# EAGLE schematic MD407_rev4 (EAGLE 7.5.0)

## Sheet 1 of 7: OVERVIEW
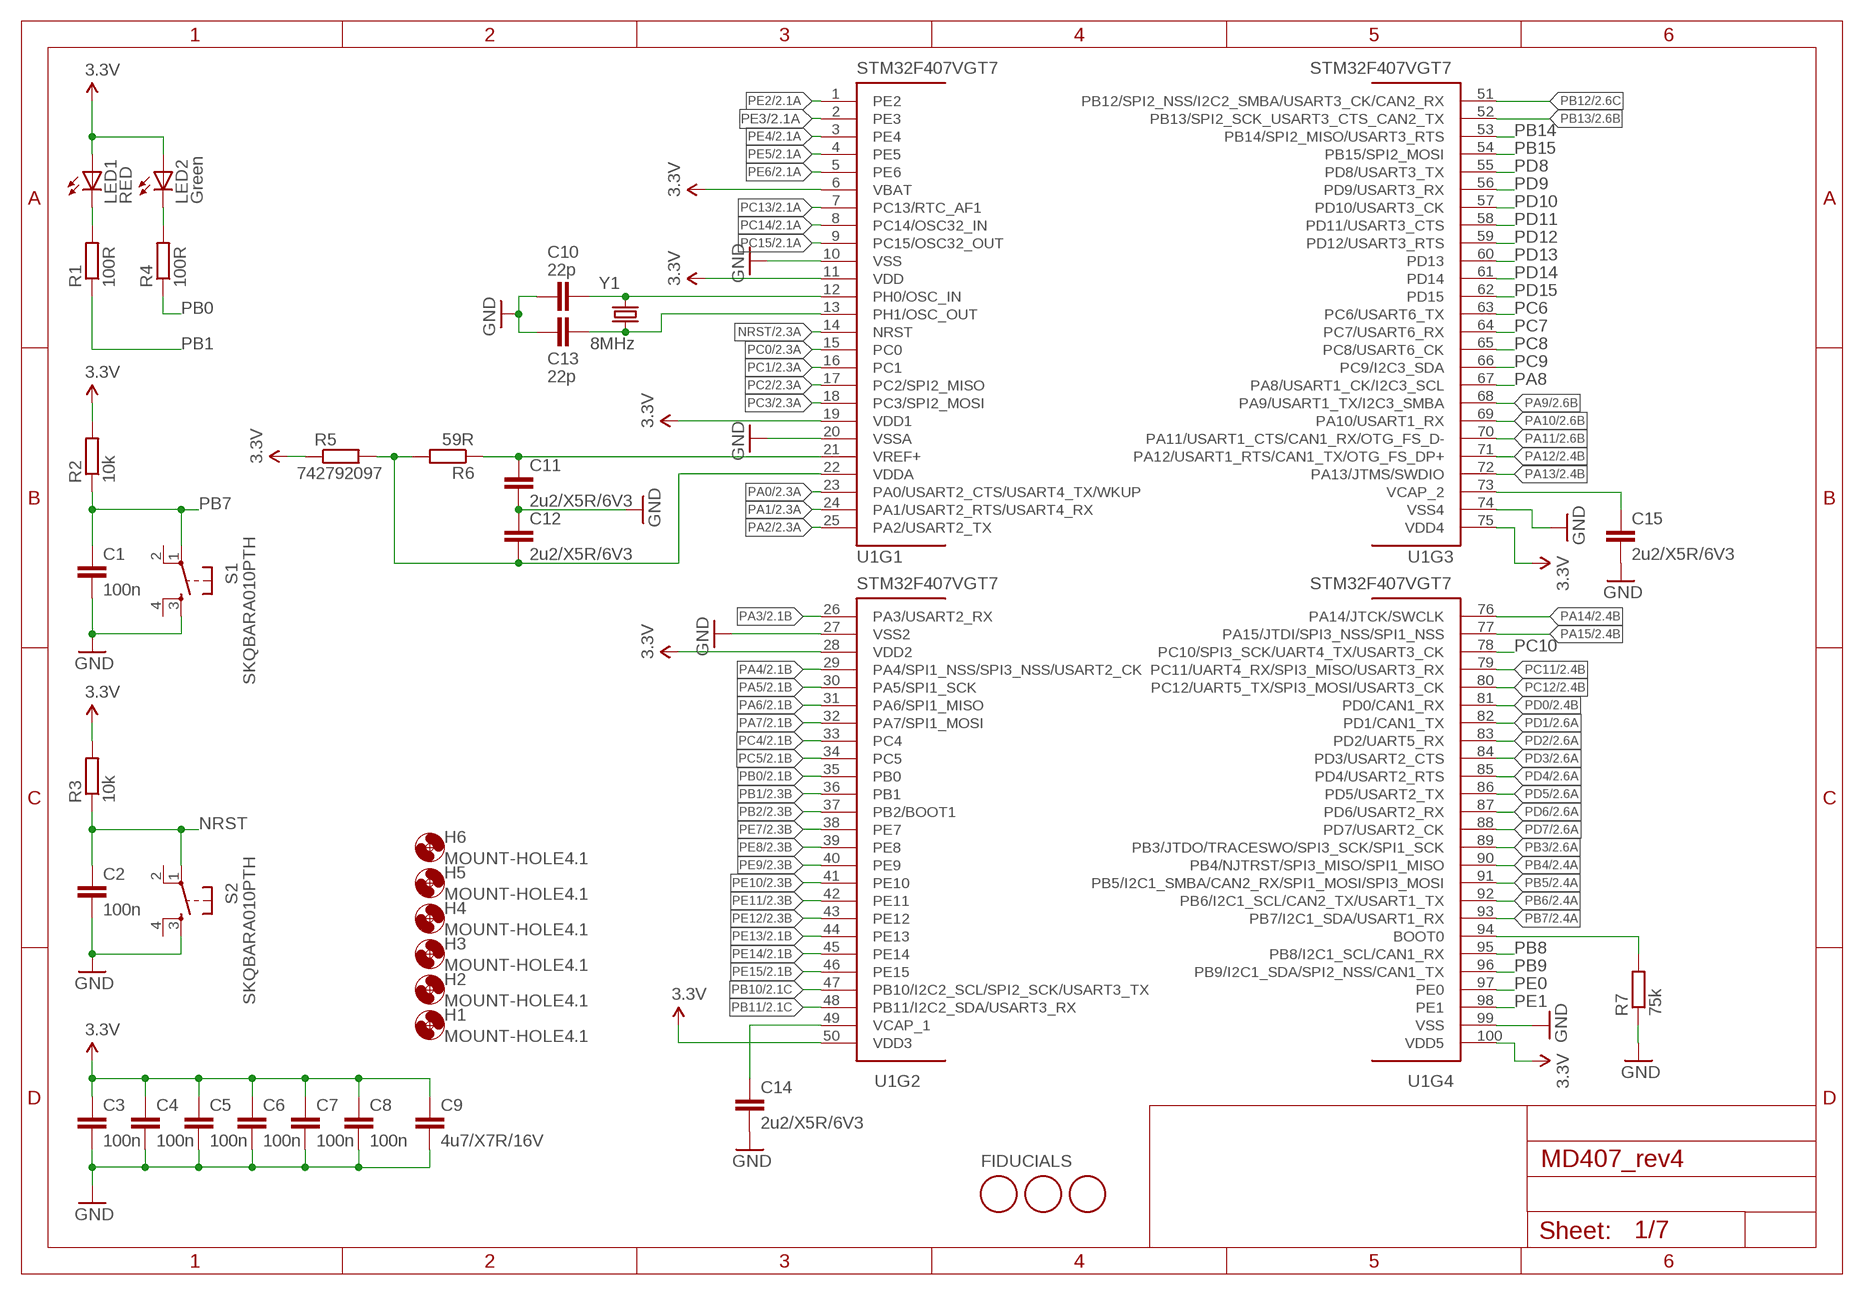
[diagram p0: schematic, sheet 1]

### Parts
C1  100n  C-EUC0603  [C0603]
C2  100n  C-EUC0603  [C0603]
C3  100n  C-EUC0603  [C0603]
C4  100n  C-EUC0603  [C0603]
C5  100n  C-EUC0603  [C0603]
C6  100n  C-EUC0603  [C0603]
C7  100n  C-EUC0603  [C0603]
C8  100n  C-EUC0603  [C0603]
C9  4u7/X7R/16V  C-EUC0805  [C0805]
C10  22p  C-EUC0603  [C0603]
C11  2u2/X5R/6V3  C-EUC0603  [C0603]
C12  2u2/X5R/6V3  C-EUC0603  [C0603]
C13  22p  C-EUC0603  [C0603]
C14  2u2/X5R/6V3  C-EUC0603  [C0603]
C15  2u2/X5R/6V3  C-EUC0603  [C0603]
H1  MOUNT-HOLE4.1  [4,1]
H2  MOUNT-HOLE4.1  [4,1]
H3  MOUNT-HOLE4.1  [4,1]
H4  MOUNT-HOLE4.1  [4,1]
H5  MOUNT-HOLE4.1  [4,1]
H6  MOUNT-HOLE4.1  [4,1]
LED1  RED  LED0603  [LED-0603]
LED2  Green  LED0603  [LED-0603]
R1  100R  R-EU_R0603  [R0603]
R2  10k  R-EU_R0603  [R0603]
R3  10k  R-EU_R0603  [R0603]
R4  100R  R-EU_R0603  [R0603]
R5  742792097  R-EU_R0805  [R0805]
R6  59R  R-EU_R0603  [R0603]
R7  75k  R-EU_R0603  [R0603]
S1  SKQBARA010PTH  [TACTILE-PTH]
S2  SKQBARA010PTH  [TACTILE-PTH]
U1  STM32F407VGT7  [LQFP100]
U$1  FIDUCIAL  [FIDUCIAL_1MM]
U$2  FIDUCIAL  [FIDUCIAL_1MM]
U$3  FIDUCIAL  [FIDUCIAL_1MM]
Y1  8MHz  7B-8.000MAAJ-T  [CRYSTAL-SMD-5X3]

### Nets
3.3V: C3.1 C4.1 C5.1 C6.1 C7.1 C8.1 C9.1 LED1.A LED2.A R2.2 R3.2 R5.1 U1.6(VBAT) U1.11(VDD) U1.19(VDD1) U1.28(VDD2) U1.50(VDD3) U1.75(VDD4) U1.100(VDD5) ; also sheet 2,3,4,5,6,7
GND: C1.2 C2.2 C3.2 C4.2 C5.2 C6.2 C7.2 C8.2 C9.2 C10.1 C11.2 C12.1 C13.2 C14.2 C15.2 R7.1 S1.3 S2.3 U1.10(VSS) U1.20(VSSA) U1.27(VSS2) U1.74(VSS4) U1.99(VSS) ; also sheet 2,3,4,5,6,7
N$9: LED2.C R4.2
N$11: R7.2 U1.94(BOOT0)
N$27: C15.1 U1.73(VCAP_2)
N$43: C12.2 R5.2 R6.2 U1.22(VDDA)
N$45: C10.2 U1.12(PH0/OSC_IN) Y1.3
N$49: C13.1 U1.13(PH1/OSC_OUT) Y1.1
N$63: C11.1 R6.1 U1.21(VREF+)
N$77: C14.1 U1.49(VCAP_1)
N$87: LED1.C R1.2
NRST: C2.1 R3.1 S2.1 U1.14(NRST) ; also sheet 2,6
PA0: U1.23(PA0/USART2_CTS/USART4_TX/WKUP) ; also sheet 2
PA1: U1.24(PA1/USART2_RTS/USART4_RX) ; also sheet 2,6
PA2: U1.25(PA2/USART2_TX) ; also sheet 2,6
PA3: U1.26(PA3/USART2_RX) ; also sheet 2
PA4: U1.29(PA4/SPI1_NSS/SPI3_NSS/USART2_CK) ; also sheet 2
PA5: U1.30(PA5/SPI1_SCK) ; also sheet 2,3
PA6: U1.31(PA6/SPI1_MISO) ; also sheet 2
PA7: U1.32(PA7/SPI1_MOSI) ; also sheet 2,6
PA8: U1.67(PA8/USART1_CK/I2C3_SCL) ; also sheet 2
PA9: U1.68(PA9/USART1_TX/I2C3_SMBA) ; also sheet 2,4
PA10: U1.69(PA10/USART1_RX) ; also sheet 2,4
PA11: U1.70(PA11/USART1_CTS/CAN1_RX/OTG_FS_D-) ; also sheet 2,4
PA12: U1.71(PA12/USART1_RTS/CAN1_TX/OTG_FS_DP+) ; also sheet 2,4
PA13: U1.72(PA13/JTMS/SWDIO) ; also sheet 2
PA14: U1.76(PA14/JTCK/SWCLK) ; also sheet 2
PA15: U1.77(PA15/JTDI/SPI3_NSS/SPI1_NSS) ; also sheet 2
PB0: R4.1 U1.35(PB0) ; also sheet 2
PB1: R1.1 U1.36(PB1) ; also sheet 2
PB2: U1.37(PB2/BOOT1) ; also sheet 2
PB3: U1.89(PB3/JTDO/TRACESWO/SPI3_SCK/SPI1_SCK) ; also sheet 2
PB4: U1.90(PB4/NJTRST/SPI3_MISO/SPI1_MISO) ; also sheet 2
PB5: U1.91(PB5/I2C1_SMBA/CAN2_RX/SPI1_MOSI/SPI3_MOSI) ; also sheet 2,7
PB6: U1.92(PB6/I2C1_SCL/CAN2_TX/USART1_TX) ; also sheet 2,7
PB7: C1.1 R2.1 S1.1 U1.93(PB7/I2C1_SDA/USART1_RX) ; also sheet 2
PB8: U1.95(PB8/I2C1_SCL/CAN1_RX) ; also sheet 2,7
PB9: U1.96(PB9/I2C1_SDA/SPI2_NSS/CAN1_TX) ; also sheet 2,7
PB10: U1.47(PB10/I2C2_SCL/SPI2_SCK/USART3_TX) ; also sheet 2
PB11: U1.48(PB11/I2C2_SDA/USART3_RX) ; also sheet 2,6
PB12: U1.51(PB12/SPI2_NSS/I2C2_SMBA/USART3_CK/CAN2_RX) ; also sheet 2,6
PB13: U1.52(PB13/SPI2_SCK_USART3_CTS_CAN2_TX) ; also sheet 2,6
PB14: U1.53(PB14/SPI2_MISO/USART3_RTS) ; also sheet 2
PB15: U1.54(PB15/SPI2_MOSI) ; also sheet 2
PC0: U1.15(PC0) ; also sheet 2
PC1: U1.16(PC1) ; also sheet 2,6
PC2: U1.17(PC2/SPI2_MISO) ; also sheet 2
PC3: U1.18(PC3/SPI2_MOSI) ; also sheet 2
PC4: U1.33(PC4) ; also sheet 2,6
PC5: U1.34(PC5) ; also sheet 2,6
PC6: U1.63(PC6/USART6_TX) ; also sheet 2
PC7: U1.64(PC7/USART6_RX) ; also sheet 2
PC8: U1.65(PC8/USART6_CK) ; also sheet 2
PC9: U1.66(PC9/I2C3_SDA) ; also sheet 2
PC10: U1.78(PC10/SPI3_SCK/UART4_TX/USART3_CK) ; also sheet 2,3
PC11: U1.79(PC11/UART4_RX/SPI3_MISO/USART3_RX) ; also sheet 2,3
PC12: U1.80(PC12/UART5_TX/SPI3_MOSI/USART3_CK) ; also sheet 2,3
PC13: U1.7(PC13/RTC_AF1) ; also sheet 2
PC14: U1.8(PC14/OSC32_IN) ; also sheet 2
PC15: U1.9(PC15/OSC32_OUT) ; also sheet 2
PD0: U1.81(PD0/CAN1_RX) ; also sheet 2
PD1: U1.82(PD1/CAN1_TX) ; also sheet 2
PD2: U1.83(PD2/UART5_RX) ; also sheet 2
PD3: U1.84(PD3/USART2_CTS) ; also sheet 2,3
PD4: U1.85(PD4/USART2_RTS) ; also sheet 2
PD5: U1.86(PD5/USART2_TX) ; also sheet 2
PD6: U1.87(PD6/USART2_RX) ; also sheet 2
PD7: U1.88(PD7/USART2_CK) ; also sheet 2
PD8: U1.55(PD8/USART3_TX) ; also sheet 2
PD9: U1.56(PD9/USART3_RX) ; also sheet 2
PD10: U1.57(PD10/USART3_CK) ; also sheet 2
PD11: U1.58(PD11/USART3_CTS) ; also sheet 2
PD12: U1.59(PD12/USART3_RTS) ; also sheet 2
PD13: U1.60(PD13) ; also sheet 2
PD14: U1.61(PD14) ; also sheet 2
PD15: U1.62(PD15) ; also sheet 2
PE0: U1.97(PE0) ; also sheet 2
PE1: U1.98(PE1) ; also sheet 2
PE2: U1.1(PE2) ; also sheet 2
PE3: U1.2(PE3) ; also sheet 2
PE4: U1.3(PE4) ; also sheet 2
PE5: U1.4(PE5) ; also sheet 2
PE6: U1.5(PE6) ; also sheet 2
PE7: U1.38(PE7) ; also sheet 2
PE8: U1.39(PE8) ; also sheet 2
PE9: U1.40(PE9) ; also sheet 2
PE10: U1.41(PE10) ; also sheet 2
PE11: U1.42(PE11) ; also sheet 2
PE12: U1.43(PE12) ; also sheet 2
PE13: U1.44(PE13) ; also sheet 2
PE14: U1.45(PE14) ; also sheet 2
PE15: U1.46(PE15) ; also sheet 2
Unconnected: S1.2 S1.4 S2.2 S2.4

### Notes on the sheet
- FIDUCIALS

## Sheet 2 of 7: EXP-headers
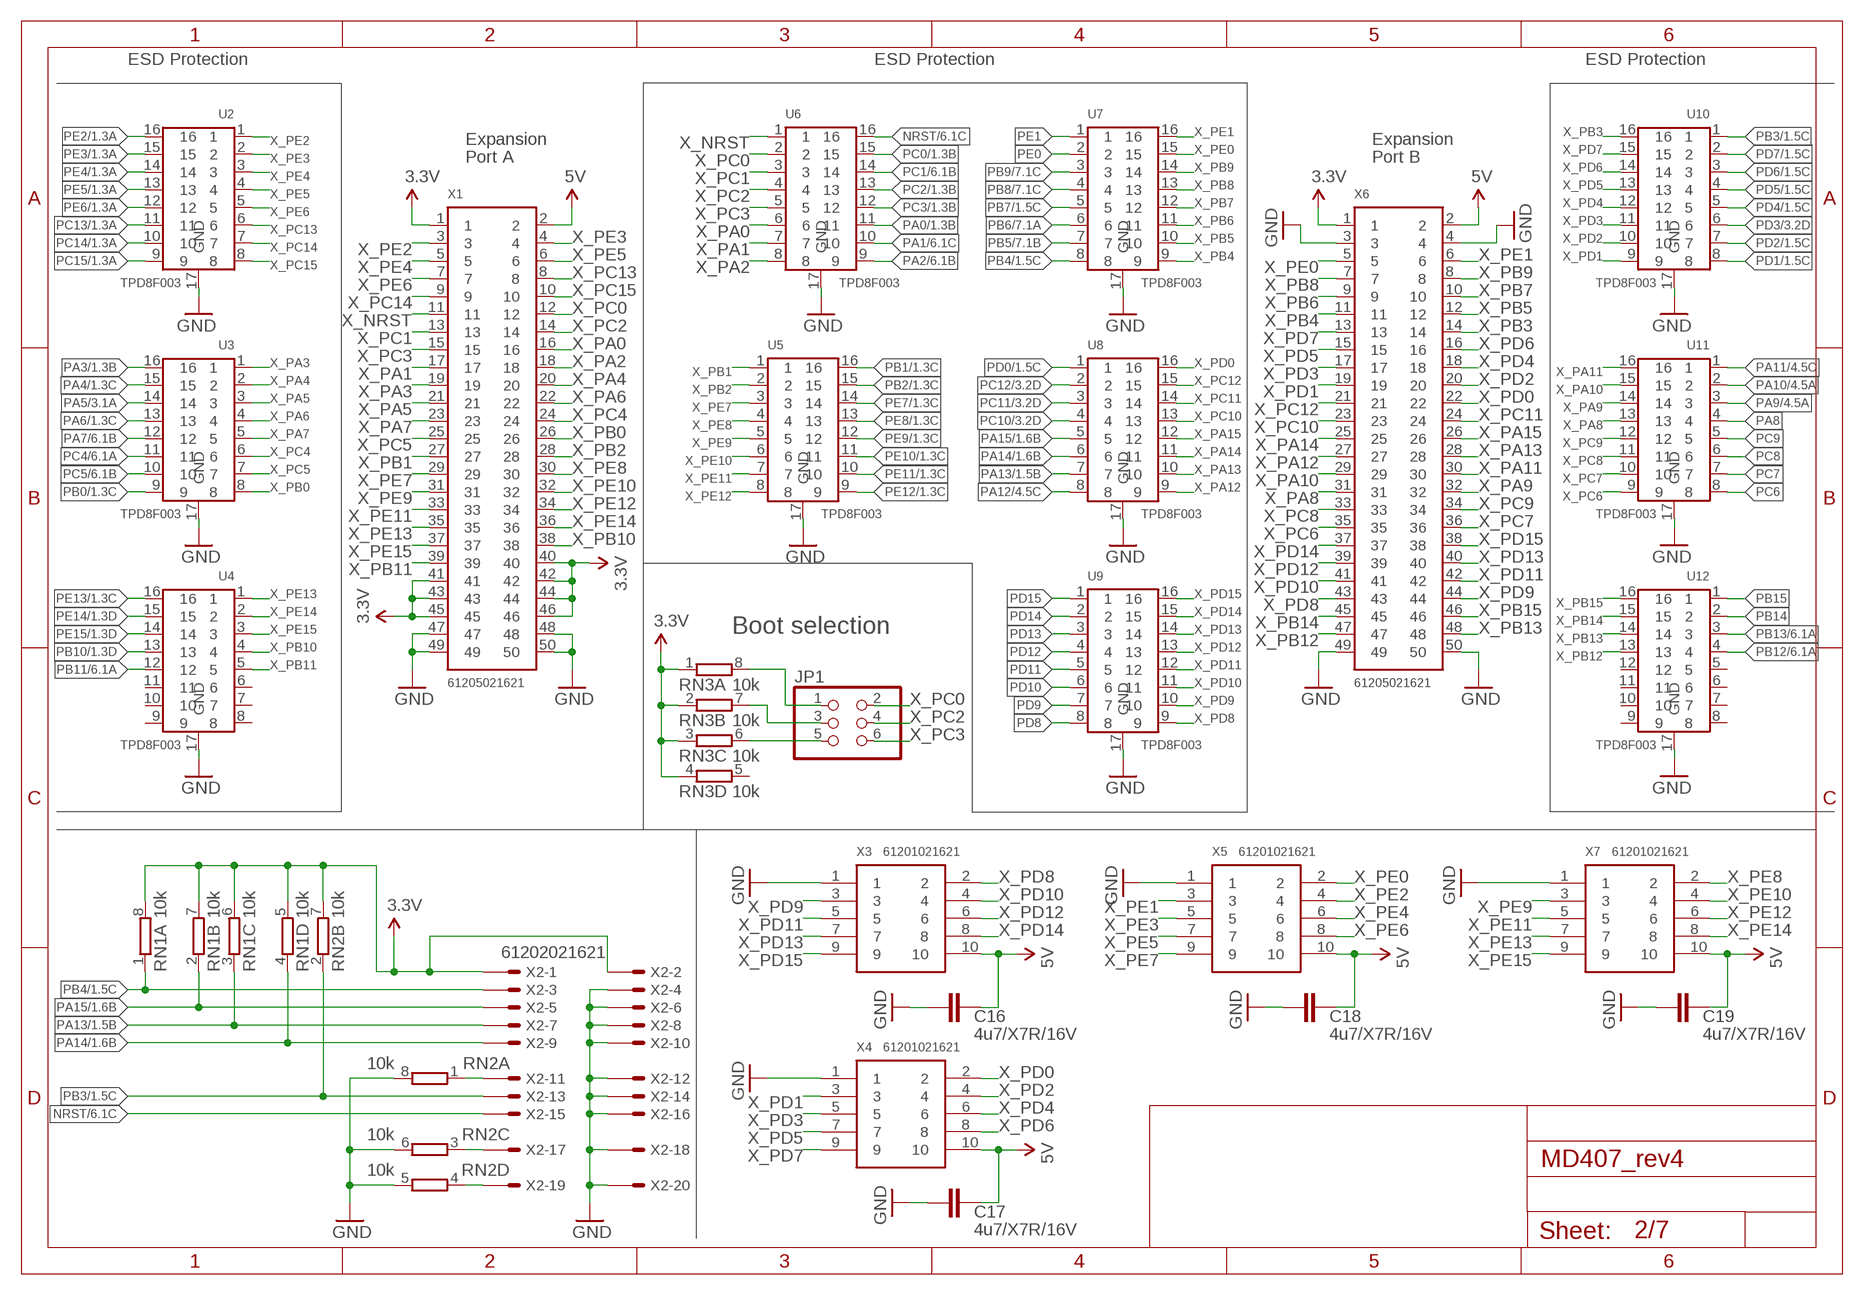
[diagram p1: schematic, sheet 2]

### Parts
C16  4u7/X7R/16V  C-EUC0805  [C0805]
C17  4u7/X7R/16V  C-EUC0805  [C0805]
C18  4u7/X7R/16V  C-EUC0805  [C0805]
C19  4u7/X7R/16V  C-EUC0805  [C0805]
JP1  PINHD-2X3  [2X03]
RN1  10k  4R-NCAY16  [CAY16]
RN2  10k  4R-NCAY16  [CAY16]
RN3  10k  4R-NCAY16  [CAY16]
U2  TPD8F003  [16-WFDFN]
U3  TPD8F003  [16-WFDFN]
U4  TPD8F003  [16-WFDFN]
U5  TPD8F003  [16-WFDFN]
U6  TPD8F003  [16-WFDFN]
U7  TPD8F003  [16-WFDFN]
U8  TPD8F003  [16-WFDFN]
U9  TPD8F003  [16-WFDFN]
U10  TPD8F003  [16-WFDFN]
U11  TPD8F003  [16-WFDFN]
U12  TPD8F003  [16-WFDFN]
X1  61205021621  [057-050-1]
X2  61202021621  [057-020-1]
X3  61201021621  [057-010-1]
X4  61201021621  [057-010-1]
X5  61201021621  [057-010-1]
X6  61205021621  [057-050-1]
X7  61201021621  [057-010-1]

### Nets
3.3V: RN1.5 RN1.6 RN1.7 RN1.8 RN2.7 RN3.1 RN3.2 RN3.3 RN3.4 X1.1 X1.40 X1.41 X1.42 X1.43 X1.44 X1.45 X1.46 X2.1 X2.2 X6.1 ; also sheet 1,3,4,5,6,7
5V: C16.1 C17.1 C18.1 C19.1 X1.2 X3.10 X4.10 X5.10 X6.2 X7.10 ; also sheet 3,4,5,7
GND: C16.2 C17.2 C18.2 C19.2 RN2.5 RN2.6 RN2.8 U2.17(GND) U3.17(GND) U4.17(GND) U5.17(GND) U6.17(GND) U7.17(GND) U8.17(GND) U9.17(GND) U10.17(GND) U11.17(GND) U12.17(GND) X1.47 X1.48 X1.49 X1.50 X2.4 X2.6 X2.8 X2.10 X2.12 X2.14 X2.16 X2.18 X2.20 X3.1 X4.1 X5.1 X6.3 X6.4 X6.49 X6.50 X7.1 ; also sheet 1,3,4,5,6,7
N$8: JP1.1 RN3.8
N$23: JP1.3 RN3.7
N$41: JP1.5 RN3.6
N$71: RN2.3 X2.17
N$96: RN2.4 X2.19
N$97: RN2.1 X2.11
NRST: U6.16 X2.15 ; also sheet 1,6
PA0: U6.11 ; also sheet 1
PA1: U6.10 ; also sheet 1,6
PA2: U6.9 ; also sheet 1,6
PA3: U3.16 ; also sheet 1
PA4: U3.15 ; also sheet 1
PA5: U3.14 ; also sheet 1,3
PA6: U3.13 ; also sheet 1
PA7: U3.12 ; also sheet 1,6
PA8: U11.4 ; also sheet 1
PA9: U11.3 ; also sheet 1,4
PA10: U11.2 ; also sheet 1,4
PA11: U11.1 ; also sheet 1,4
PA12: U8.8 ; also sheet 1,4
PA13: RN1.3 U8.7 X2.7 ; also sheet 1
PA14: RN1.4 U8.6 X2.9 ; also sheet 1
PA15: RN1.2 U8.5 X2.5 ; also sheet 1
PB0: U3.9 ; also sheet 1
PB1: U5.16 ; also sheet 1
PB2: U5.15 ; also sheet 1
PB3: RN2.2 U10.1 X2.13 ; also sheet 1
PB4: RN1.1 U7.8 X2.3 ; also sheet 1
PB5: U7.7 ; also sheet 1,7
PB6: U7.6 ; also sheet 1,7
PB7: U7.5 ; also sheet 1
PB8: U7.4 ; also sheet 1,7
PB9: U7.3 ; also sheet 1,7
PB10: U4.13 ; also sheet 1
PB11: U4.12 ; also sheet 1,6
PB12: U12.4 ; also sheet 1,6
PB13: U12.3 ; also sheet 1,6
PB14: U12.2 ; also sheet 1
PB15: U12.1 ; also sheet 1
PC0: U6.15 ; also sheet 1
PC1: U6.14 ; also sheet 1,6
PC2: U6.13 ; also sheet 1
PC3: U6.12 ; also sheet 1
PC4: U3.11 ; also sheet 1,6
PC5: U3.10 ; also sheet 1,6
PC6: U11.8 ; also sheet 1
PC7: U11.7 ; also sheet 1
PC8: U11.6 ; also sheet 1
PC9: U11.5 ; also sheet 1
PC10: U8.4 ; also sheet 1,3
PC11: U8.3 ; also sheet 1,3
PC12: U8.2 ; also sheet 1,3
PC13: U2.11 ; also sheet 1
PC14: U2.10 ; also sheet 1
PC15: U2.9 ; also sheet 1
PD0: U8.1 ; also sheet 1
PD1: U10.8 ; also sheet 1
PD2: U10.7 ; also sheet 1
PD3: U10.6 ; also sheet 1,3
PD4: U10.5 ; also sheet 1
PD5: U10.4 ; also sheet 1
PD6: U10.3 ; also sheet 1
PD7: U10.2 ; also sheet 1
PD8: U9.8 ; also sheet 1
PD9: U9.7 ; also sheet 1
PD10: U9.6 ; also sheet 1
PD11: U9.5 ; also sheet 1
PD12: U9.4 ; also sheet 1
PD13: U9.3 ; also sheet 1
PD14: U9.2 ; also sheet 1
PD15: U9.1 ; also sheet 1
PE0: U7.2 ; also sheet 1
PE1: U7.1 ; also sheet 1
PE2: U2.16 ; also sheet 1
PE3: U2.15 ; also sheet 1
PE4: U2.14 ; also sheet 1
PE5: U2.13 ; also sheet 1
PE6: U2.12 ; also sheet 1
PE7: U5.14 ; also sheet 1
PE8: U5.13 ; also sheet 1
PE9: U5.12 ; also sheet 1
PE10: U5.11 ; also sheet 1
PE11: U5.10 ; also sheet 1
PE12: U5.9 ; also sheet 1
PE13: U4.16 ; also sheet 1
PE14: U4.15 ; also sheet 1
PE15: U4.14 ; also sheet 1
X_NRST: U6.1 X1.11
X_PA0: U6.6 X1.16
X_PA1: U6.7 X1.17
X_PA2: U6.8 X1.18
X_PA3: U3.1 X1.19
X_PA4: U3.2 X1.20
X_PA5: U3.3 X1.21
X_PA6: U3.4 X1.22
X_PA7: U3.5 X1.23
X_PA8: U11.13 X6.31
X_PA9: U11.14 X6.32
X_PA10: U11.15 X6.29
X_PA11: U11.16 X6.30
X_PA12: U8.9 X6.27
X_PA13: U8.10 X6.28
X_PA14: U8.11 X6.25
X_PA15: U8.12 X6.26
X_PB0: U3.8 X1.26
X_PB1: U5.1 X1.27
X_PB2: U5.2 X1.28
X_PB3: U10.16 X6.14
X_PB4: U7.9 X6.11
X_PB5: U7.10 X6.12
X_PB6: U7.11 X6.9
X_PB7: U7.12 X6.10
X_PB8: U7.13 X6.7
X_PB9: U7.14 X6.8
X_PB10: U4.4 X1.38
X_PB11: U4.5 X1.39
X_PB12: U12.13 X6.47
X_PB13: U12.14 X6.48
X_PB14: U12.15 X6.45
X_PB15: U12.16 X6.46
X_PC0: JP1.2 U6.2 X1.12
X_PC1: U6.3 X1.13
X_PC2: JP1.4 U6.4 X1.14
X_PC3: JP1.6 U6.5 X1.15
X_PC4: U3.6 X1.24
X_PC5: U3.7 X1.25
X_PC6: U11.9 X6.35
X_PC7: U11.10 X6.36
X_PC8: U11.11 X6.33
X_PC9: U11.12 X6.34
X_PC10: U8.13 X6.23
X_PC11: U8.14 X6.24
X_PC12: U8.15 X6.21
X_PC13: U2.6 X1.8
X_PC14: U2.7 X1.9
X_PC15: U2.8 X1.10
X_PD0: U8.16 X4.2 X6.22
X_PD1: U10.9 X4.3 X6.19
X_PD2: U10.10 X4.4 X6.20
X_PD3: U10.11 X4.5 X6.17
X_PD4: U10.12 X4.6 X6.18
X_PD5: U10.13 X4.7 X6.15
X_PD6: U10.14 X4.8 X6.16
X_PD7: U10.15 X4.9 X6.13
X_PD8: U9.9 X3.2 X6.43
X_PD9: U9.10 X3.3 X6.44
X_PD10: U9.11 X3.4 X6.41
X_PD11: U9.12 X3.5 X6.42
X_PD12: U9.13 X3.6 X6.39
X_PD13: U9.14 X3.7 X6.40
X_PD14: U9.15 X3.8 X6.37
X_PD15: U9.16 X3.9 X6.38
X_PE0: U7.15 X5.2 X6.5
X_PE1: U7.16 X5.3 X6.6
X_PE2: U2.1 X1.3 X5.4
X_PE3: U2.2 X1.4 X5.5
X_PE4: U2.3 X1.5 X5.6
X_PE5: U2.4 X1.6 X5.7
X_PE6: U2.5 X1.7 X5.8
X_PE7: U5.3 X1.29 X5.9
X_PE8: U5.4 X1.30 X7.2
X_PE9: U5.5 X1.31 X7.3
X_PE10: U5.6 X1.32 X7.4
X_PE11: U5.7 X1.33 X7.5
X_PE12: U5.8 X1.34 X7.6
X_PE13: U4.1 X1.35 X7.7
X_PE14: U4.2 X1.36 X7.8
X_PE15: U4.3 X1.37 X7.9
Unconnected: RN3.5 U4.6 U4.7 U4.8 U4.9 U4.10 U4.11 U12.5 U12.6 U12.7 U12.8 U12.9 U12.10 U12.11 U12.12

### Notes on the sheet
- ESD Protection | ESD Protection | ESD Protection
- Expansion | Expansion
- Port A | Port B
- Boot selection

## Sheet 3 of 7: SOUND + JTAG
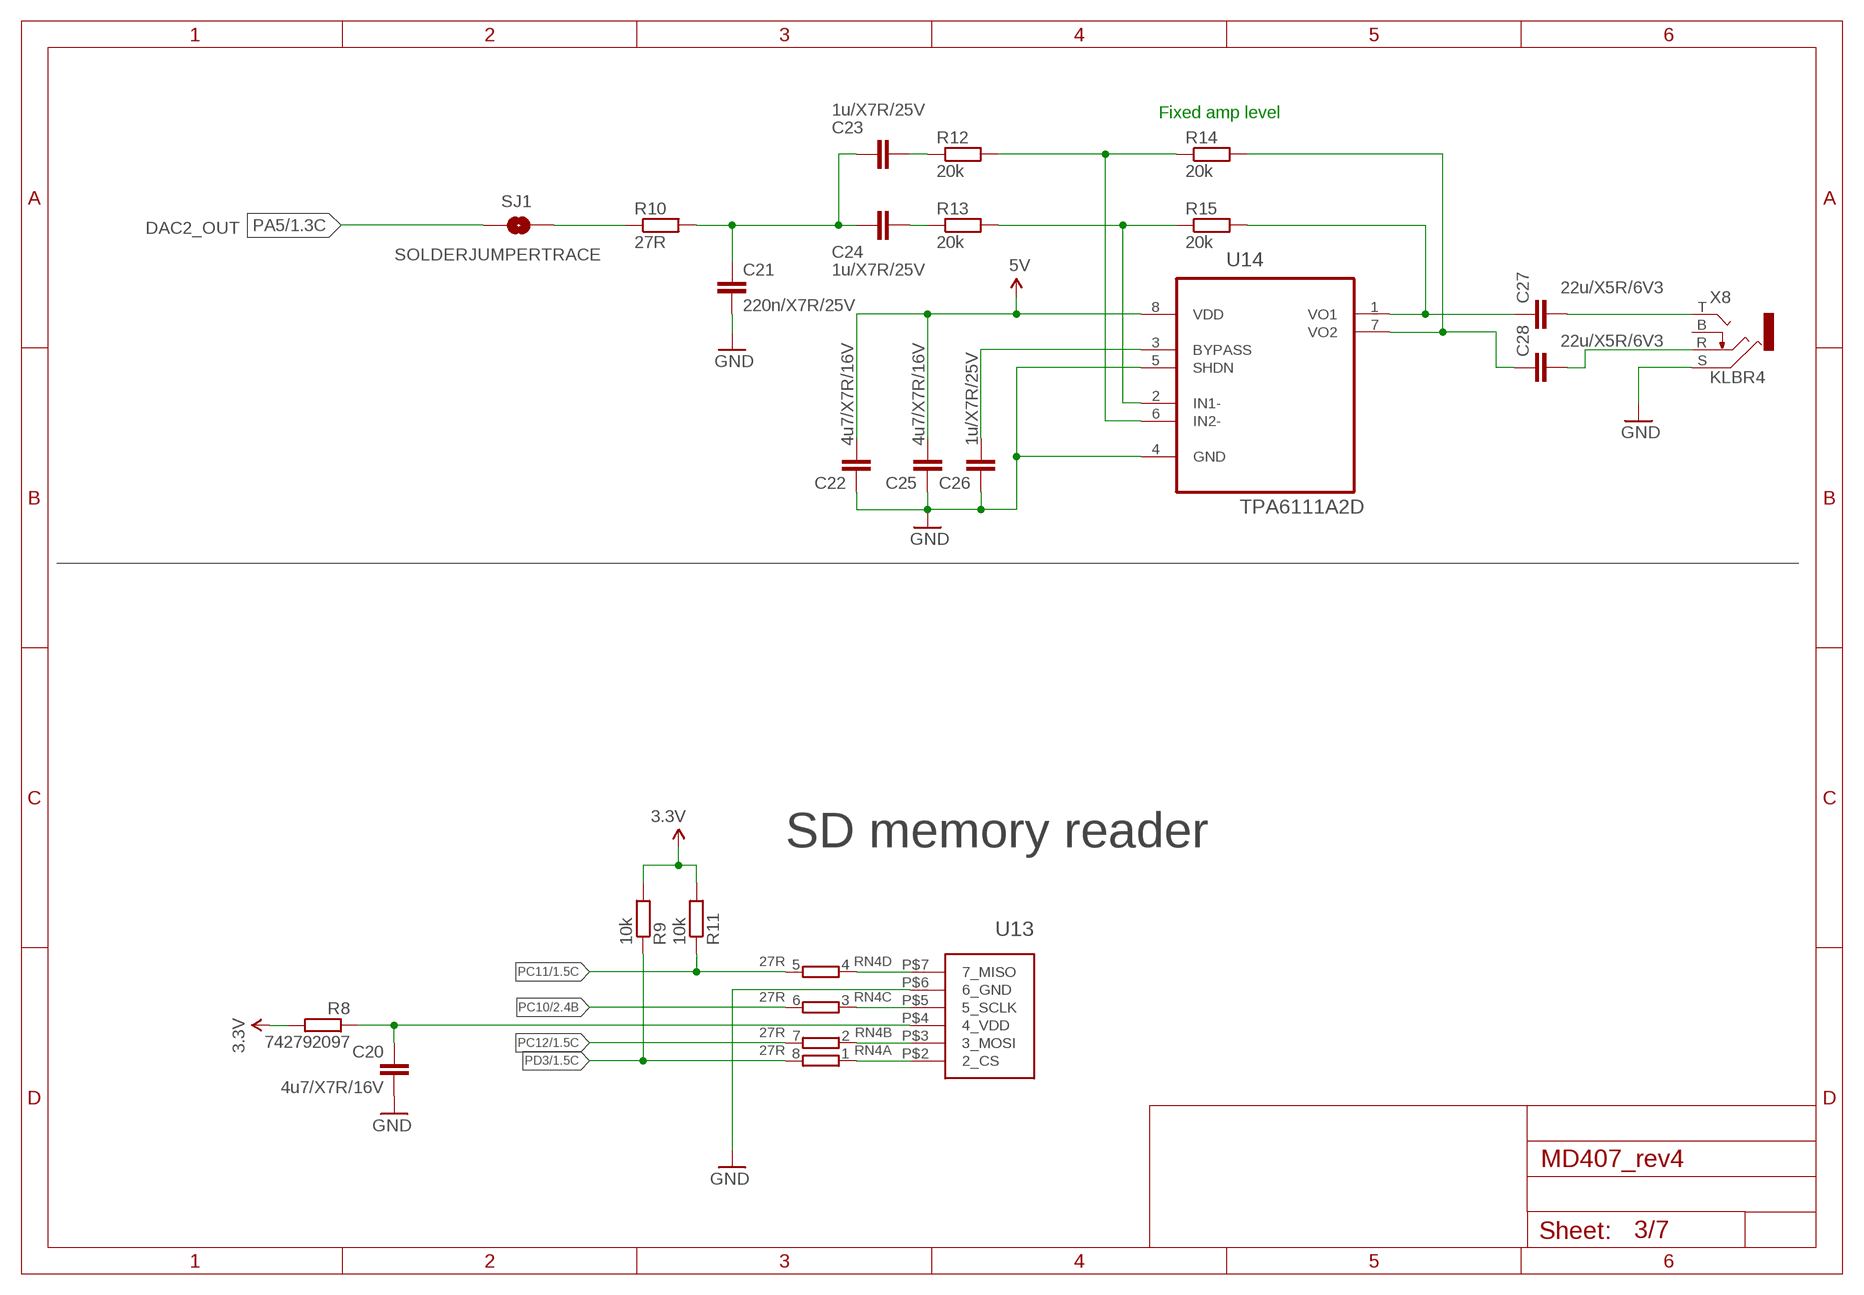
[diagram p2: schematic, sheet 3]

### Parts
C20  4u7/X7R/16V  C-EUC0805  [C0805]
C21  220n/X7R/25V  C-EUC0805  [C0805]
C22  4u7/X7R/16V  C-EUC0805  [C0805]
C23  1u/X7R/25V  C-EUC0805  [C0805]
C24  1u/X7R/25V  C-EUC0805  [C0805]
C25  4u7/X7R/16V  C-EUC0805  [C0805]
C26  1u/X7R/25V  C-EUC0805  [C0805]
C27  22u/X5R/6V3  C-EUC1206  [C1206]
C28  22u/X5R/6V3  C-EUC1206  [C1206]
R8  742792097  R-EU_R0805  [R0805]
R9  10k  R-EU_R0603  [R0603]
R10  27R  R-EU_R0603  [R0603]
R11  10k  R-EU_R0603  [R0603]
R12  20k  R-EU_R0603  [R0603]
R13  20k  R-EU_R0603  [R0603]
R14  20k  R-EU_R0603  [R0603]
R15  20k  R-EU_R0603  [R0603]
RN4  27R  4R-NCAY16  [CAY16]
SJ1  SOLDERJUMPERTRACE  [SJ_2S-TRACE]
U13  500901-0801  [MICROSD_500901-0801]
U14  TPA6111A2D  [SOIC127P600X175-8N]
X8  KLBR4  [KLBR4]

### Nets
3.3V: R8.2 R9.2 R11.2 ; also sheet 1,2,4,5,6,7
5V: C22.2 C25.2 U14.8(VDD) ; also sheet 2,4,5,7
GND: C20.2 C21.2 C22.1 C25.1 C26.1 U13.P$6(6_GND) U14.4(GND) U14.5(SHDN) X8.S ; also sheet 1,2,4,5,6,7
N$25: C27.1 R15.2 U14.1(VO1)
N$40: C20.1 R8.1 U13.P$4(4_VDD)
N$42: R12.2 R14.1 U14.6(IN2-)
N$44: RN4.1 U13.P$2(2_CS)
N$46: RN4.2 U13.P$3(3_MOSI)
N$48: R10.1 SJ1.2
N$61: RN4.3 U13.P$5(5_SCLK)
N$62: RN4.4 U13.P$7(7_MISO)
N$70: C23.2 R12.1
N$84: R13.2 R15.1 U14.2(IN1-)
N$104: C21.1 C23.1 C24.1 R10.2
N$105: C24.2 R13.1
N$106: C26.2 U14.3(BYPASS)
N$109: C28.1 R14.2 U14.7(VO2)
N$110: C27.2 X8.T
N$111: C28.2 X8.R
PA5: SJ1.1 ; also sheet 1,2
PC10: RN4.6 ; also sheet 1,2
PC11: R11.1 RN4.5 ; also sheet 1,2
PC12: RN4.7 ; also sheet 1,2
PD3: R9.1 RN4.8 ; also sheet 1,2
Unconnected: X8.B

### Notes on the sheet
- Fixed amp level
- DAC2_OUT
- SD memory reader

## Sheet 4 of 7: USB
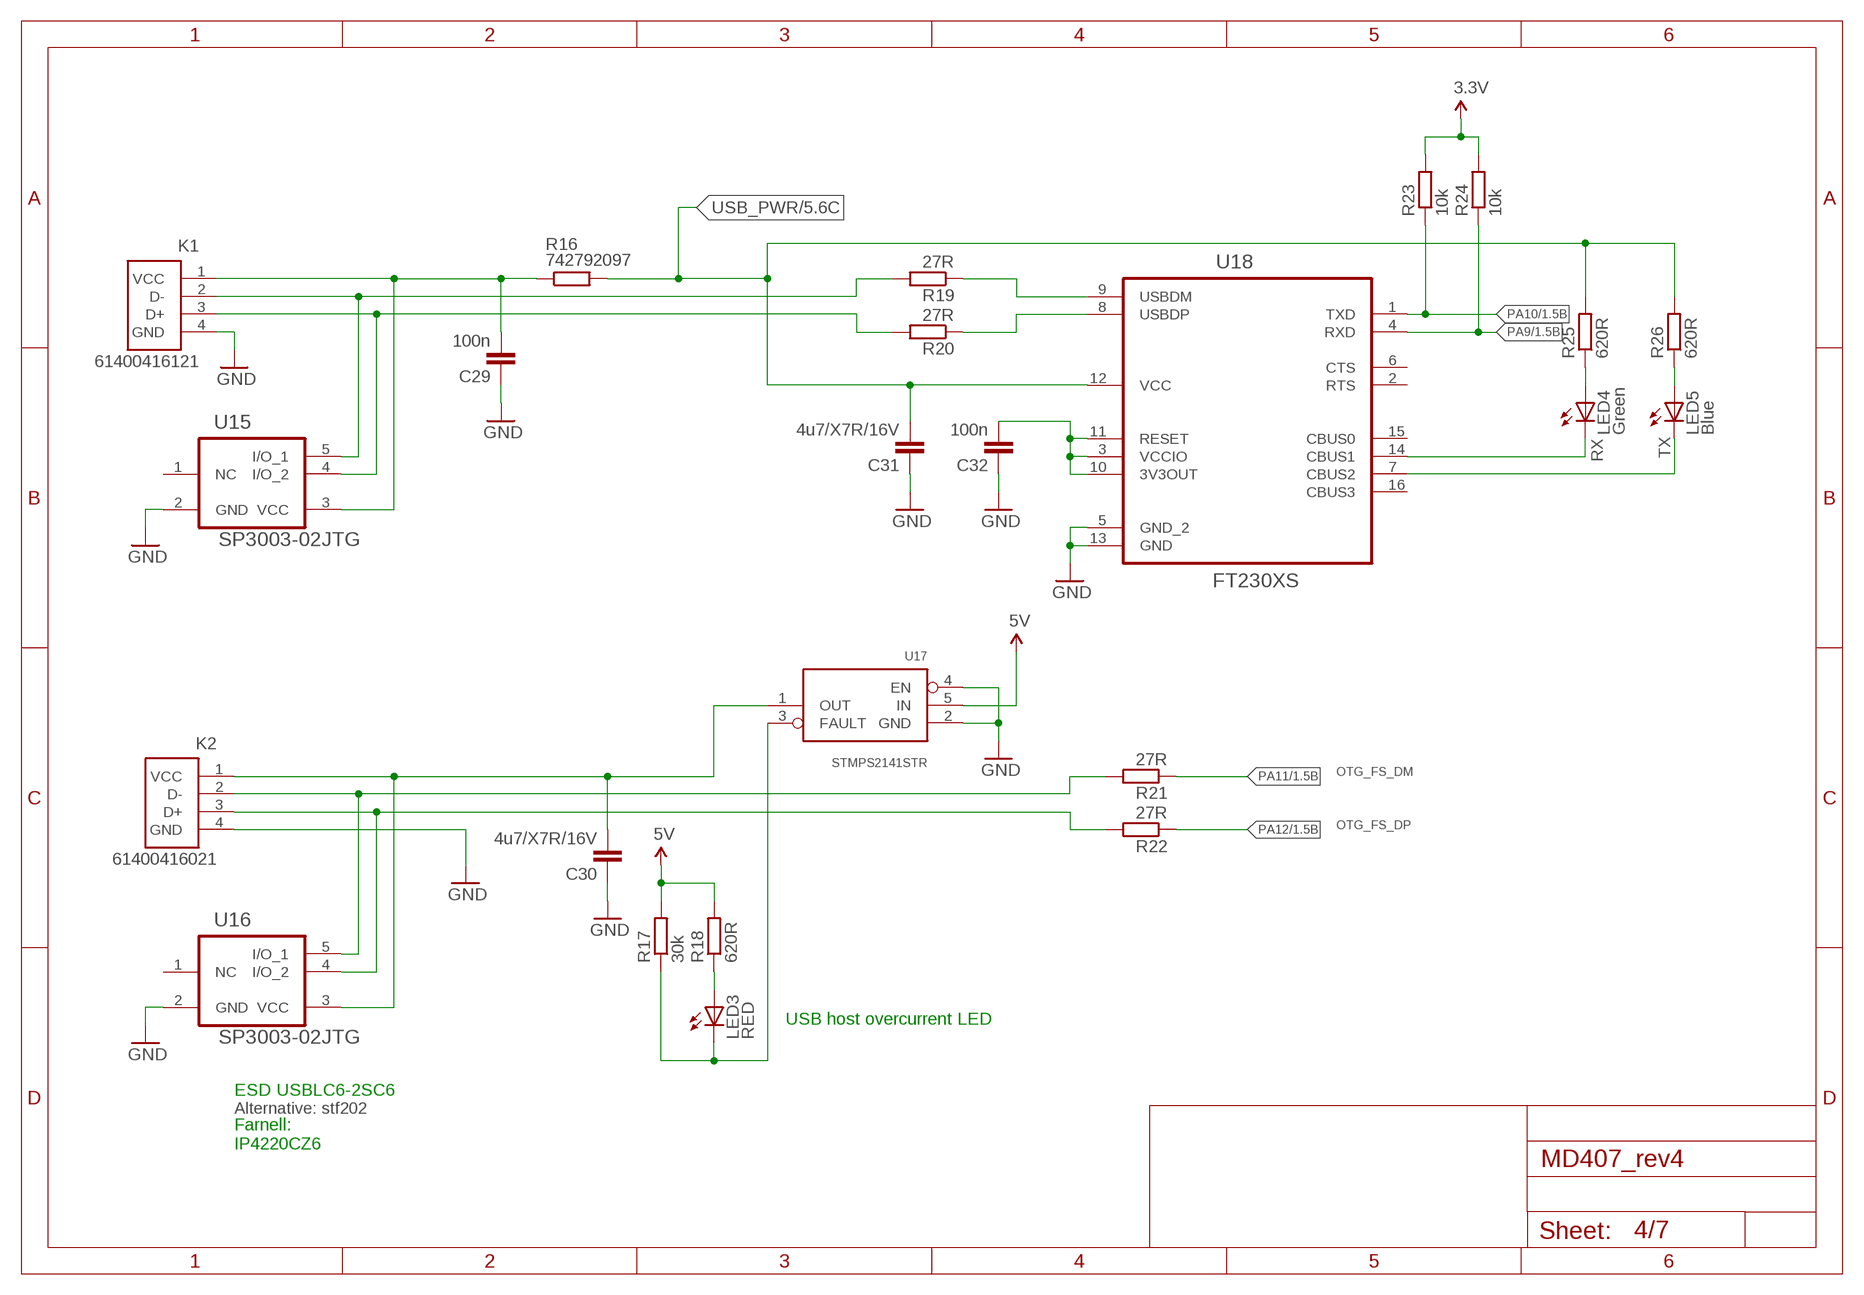
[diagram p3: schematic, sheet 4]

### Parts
C29  100n  C-EUC0603  [C0603]
C30  4u7/X7R/16V  C-EUC0805  [C0805]
C31  4u7/X7R/16V  C-EUC0805  [C0805]
C32  100n  C-EUC0603  [C0603]
K1  61400416121  [61400416121]
K2  61400416021  [61400416021]
LED3  RED  LED0603  [LED-0603]
LED4  Green  LED0603  [LED-0603]
LED5  Blue  LED0603  [LED-0603]
R16  742792097  R-EU_R0805  [R0805]
R17  30k  R-EU_R0603  [R0603]
R18  620R  R-EU_R0603  [R0603]
R19  27R  R-EU_R0603  [R0603]
R20  27R  R-EU_R0603  [R0603]
R21  27R  R-EU_R0603  [R0603]
R22  27R  R-EU_R0603  [R0603]
R23  10k  R-EU_R0603  [R0603]
R24  10k  R-EU_R0603  [R0603]
R25  620R  R-EU_R0603  [R0603]
R26  620R  R-EU_R0603  [R0603]
U15  SP3003-02JTG  [SOT65P220X110-5N]
U16  SP3003-02JTG  [SOT65P220X110-5N]
U17  STMPS2141STR  [SOT23-5]
U18  FT230XS  [SOP63P600X175-16N]

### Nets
3.3V: R23.2 R24.2 ; also sheet 1,2,3,5,6,7
5V: R17.2 R18.2 U17.5(IN) ; also sheet 2,3,5,7
GND: C29.1 C30.1 C31.1 C32.1 K1.4(GND) K2.4(GND) U15.2(GND) U16.2(GND) U17.2(GND) U17.4(EN) U18.5(GND_2) U18.13(GND) ; also sheet 1,2,3,5,6,7
N$2: R19.1 U18.9(USBDM)
N$5: LED4.A R25.1
N$13: R20.1 U18.8(USBDP)
N$15: LED5.A R26.1
N$16: K1.2(D-) R19.2 U15.5(I/O_1)
N$17: LED4.C U18.14(CBUS1)
N$18: K2.2(D-) R21.2 U16.5(I/O_1)
N$19: K2.3(D+) R22.2 U16.4(I/O_2)
N$20: K1.3(D+) R20.2 U15.4(I/O_2)
N$21: LED3.A R18.1
N$22: LED5.C U18.7(CBUS2)
N$24: LED3.C R17.1 U17.3(FAULT)
N$28: C32.2 U18.3(VCCIO) U18.10(3V3OUT) U18.11(RESET)
N$30: C30.2 K2.1(VCC) U16.3(VCC) U17.1(OUT)
N$69: C29.2 K1.1(VCC) R16.1 U15.3(VCC)
PA9: R24.1 U18.4(RXD) ; also sheet 1,2
PA10: R23.1 U18.1(TXD) ; also sheet 1,2
PA11: R21.1 ; also sheet 1,2
PA12: R22.1 ; also sheet 1,2
USB_PWR: C31.2 R16.2 R25.2 R26.2 U18.12(VCC) ; also sheet 5
Unconnected: U15.1(NC) U16.1(NC) U18.2(RTS) U18.6(CTS) U18.15(CBUS0) U18.16(CBUS3)

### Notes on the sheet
- RX | TX
- OTG_FS_DM
- OTG_FS_DP
- USB host overcurrent LED
- ESD USBLC6-2SC6
- Alternative: stf202
- Farnell:
  IP4220CZ6

## Sheet 5 of 7: PWR
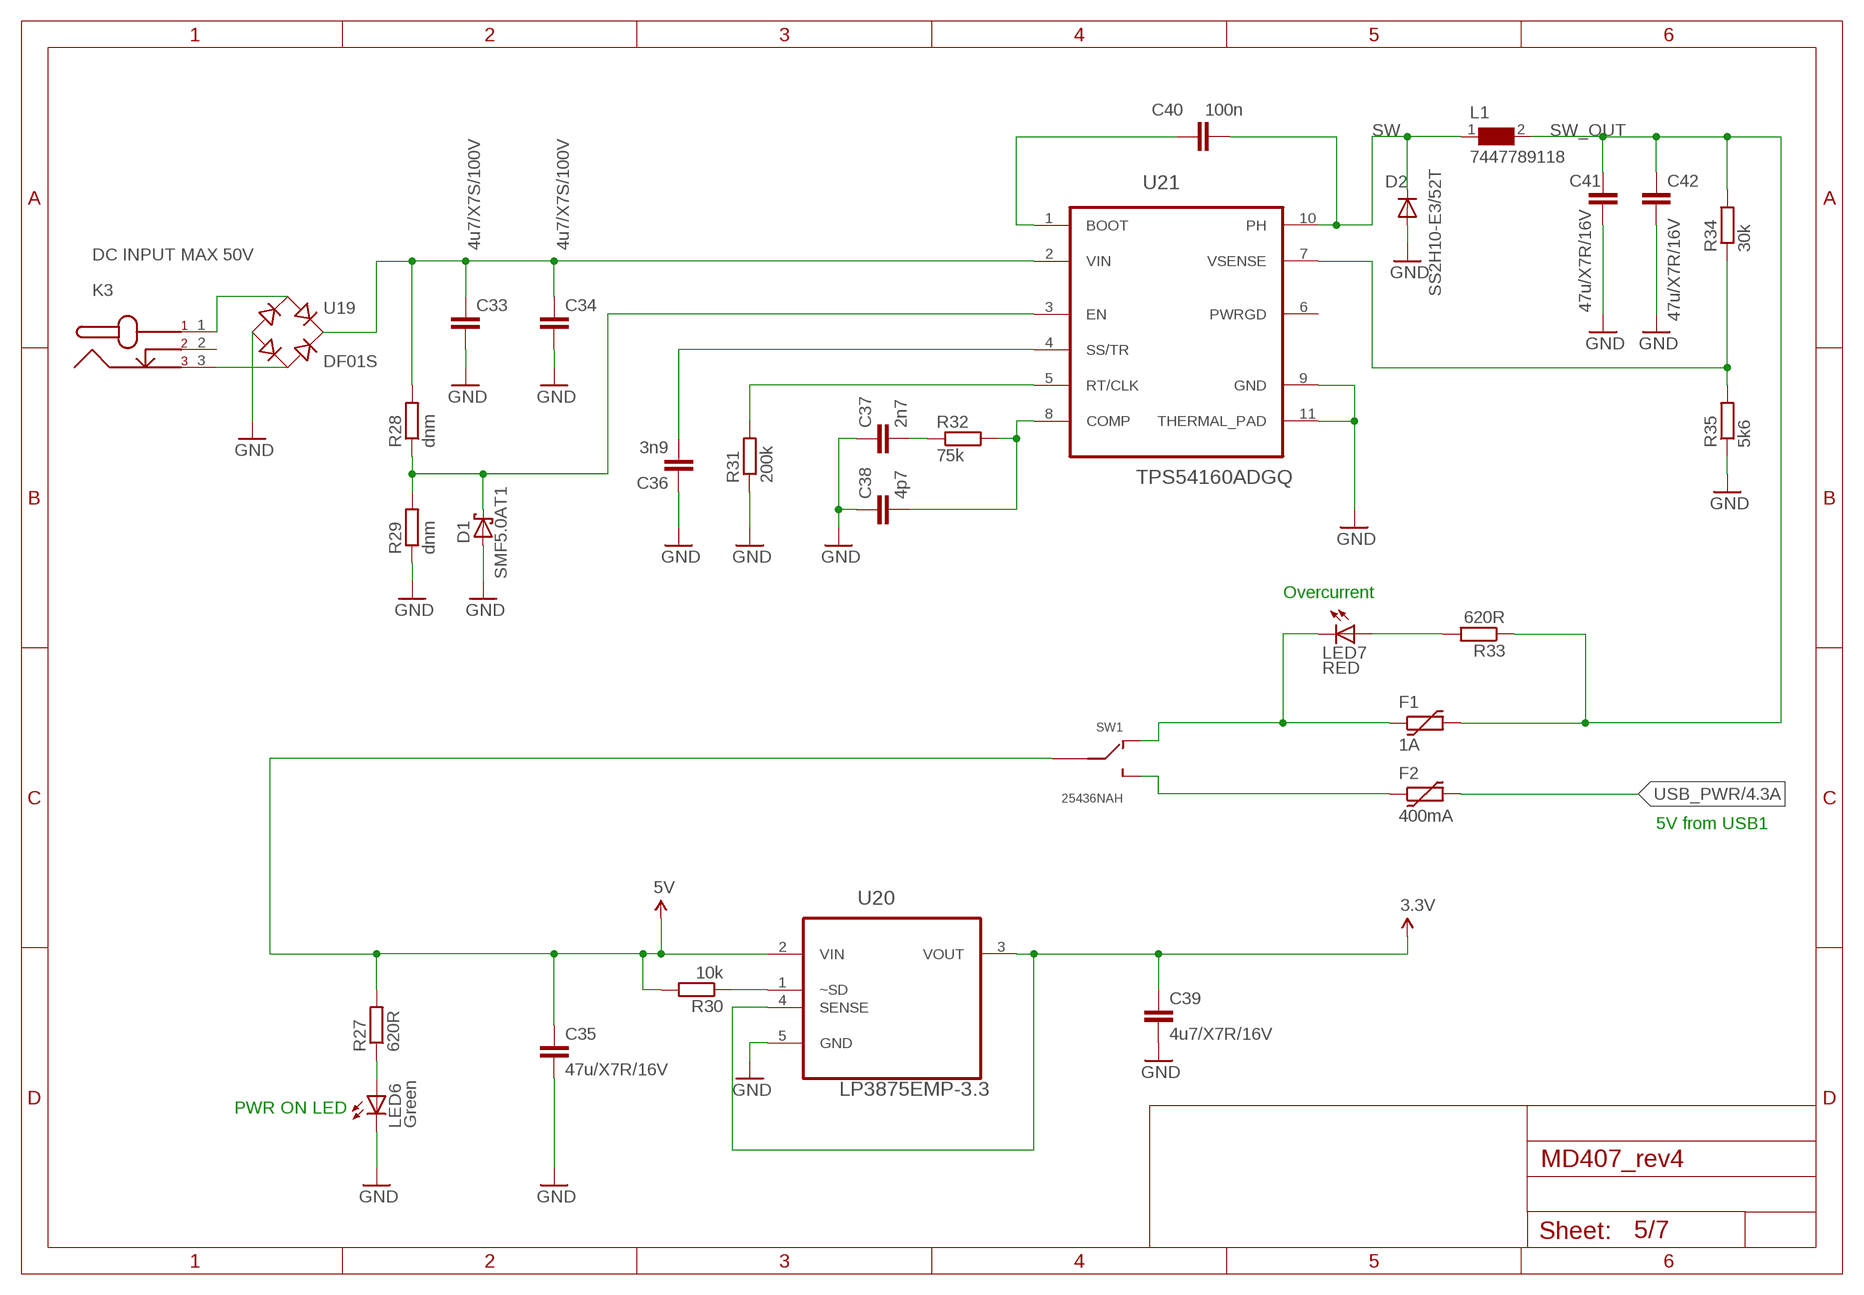
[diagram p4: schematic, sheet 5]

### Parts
C33  4u7/X7S/100V  C-EUC1210  [C1210]
C34  4u7/X7S/100V  C-EUC1210  [C1210]
C35  47u/X7R/16V  C-EUC2220K  [C2220K]
C36  3n9  C-EUC0603  [C0603]
C37  2n7  C-EUC0603  [C0603]
C38  4p7  C-EUC0603  [C0603]
C39  4u7/X7R/16V  C-EUC0805  [C0805]
C40  100n  C-EUC0603  [C0603]
C41  47u/X7R/16V  C-EUC2220K  [C2220K]
C42  47u/X7R/16V  C-EUC2220K  [C2220K]
D1  SMF5.0AT1  [SOD123FL]
D2  SS2H10-E3/52T  DIODE-DO214AA  [DO214AA]
F1  1A  1812L050PR  [PTC1812L]
F2  400mA  1812L020PR  [PTC1812L]
K3  FC681465P  [DC-PLUG]
L1  7447789118  WE-PD-7447789118_7332/7345_PLASTIC_BASE  [WE-PD_7332/7345_PLASTIC_BASE]
LED6  Green  LED0603  [LED-0603]
LED7  RED  LED0603  [LED-0603]
R27  620R  R-EU_R0603  [R0603]
R28  dnm  R-EU_R0603  [R0603]
R29  dnm  R-EU_R0603  [R0603]
R30  10k  R-EU_R0603  [R0603]
R31  200k  R-EU_R0603  [R0603]
R32  75k  R-EU_R0603  [R0603]
R33  620R  R-EU_R0603  [R0603]
R34  30k  R-EU_R0603  [R0603]
R35  5k6  R-EU_R0603  [R0603]
SW1  25436NAH  [25436N]
U19  DF01S  [SOT508P985X260-4N]
U20  LP3875EMP-3.3  [SOT15P696X180-5N]
U21  TPS54160ADGQ  [SOP50P490X110-11N]

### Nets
3.3V: C39.1 U20.3(VOUT) U20.4(SENSE) ; also sheet 1,2,3,4,6,7
5V: C35.1 R27.2 R30.2 SW1.P$2 U20.2(VIN) ; also sheet 2,3,4,7
GND: C33.2 C34.2 C35.2 C36.1 C37.1 C38.1 C39.2 C41.2 C42.2 D1.A D2.A LED6.C R29.1 R31.1 R35.1 U19.2(-) U20.5(GND) U21.9(GND) U21.11(THERMAL_PAD) ; also sheet 1,2,3,4,6,7
N$1: LED7.A R33.2
N$3: LED6.A R27.1
N$4: C38.2 R32.2 U21.8(COMP)
N$6: K3.3 U19.3(AC2)
N$7: D1.C R28.1 R29.2 U21.3(EN)
N$10: R30.1 U20.1(~SD)
N$31: C37.2 R32.1
N$34: R34.1 R35.2 U21.7(VSENSE)
N$35: C40.1 U21.1(BOOT)
N$36: C33.1 C34.1 R28.2 U19.1(+) U21.2(VIN)
N$38: K3.1 U19.4(AC1)
N$47: C36.2 U21.4(SS/TR)
N$56: R31.2 U21.5(RT/CLK)
N$89: F1.1 LED7.C SW1.P$3
N$95: F2.1 SW1.P$1
SW: C40.2 D2.C L1.1 U21.10(PH)
SW_OUT: C41.1 C42.1 F1.2 L1.2 R33.1 R34.2
USB_PWR: F2.2 ; also sheet 4
Unconnected: K3.2 U21.6(PWRGD)

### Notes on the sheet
- DC INPUT MAX 50V
- Overcurrent
- 5V from USB1
- PWR ON LED

## Sheet 6 of 7: LAN
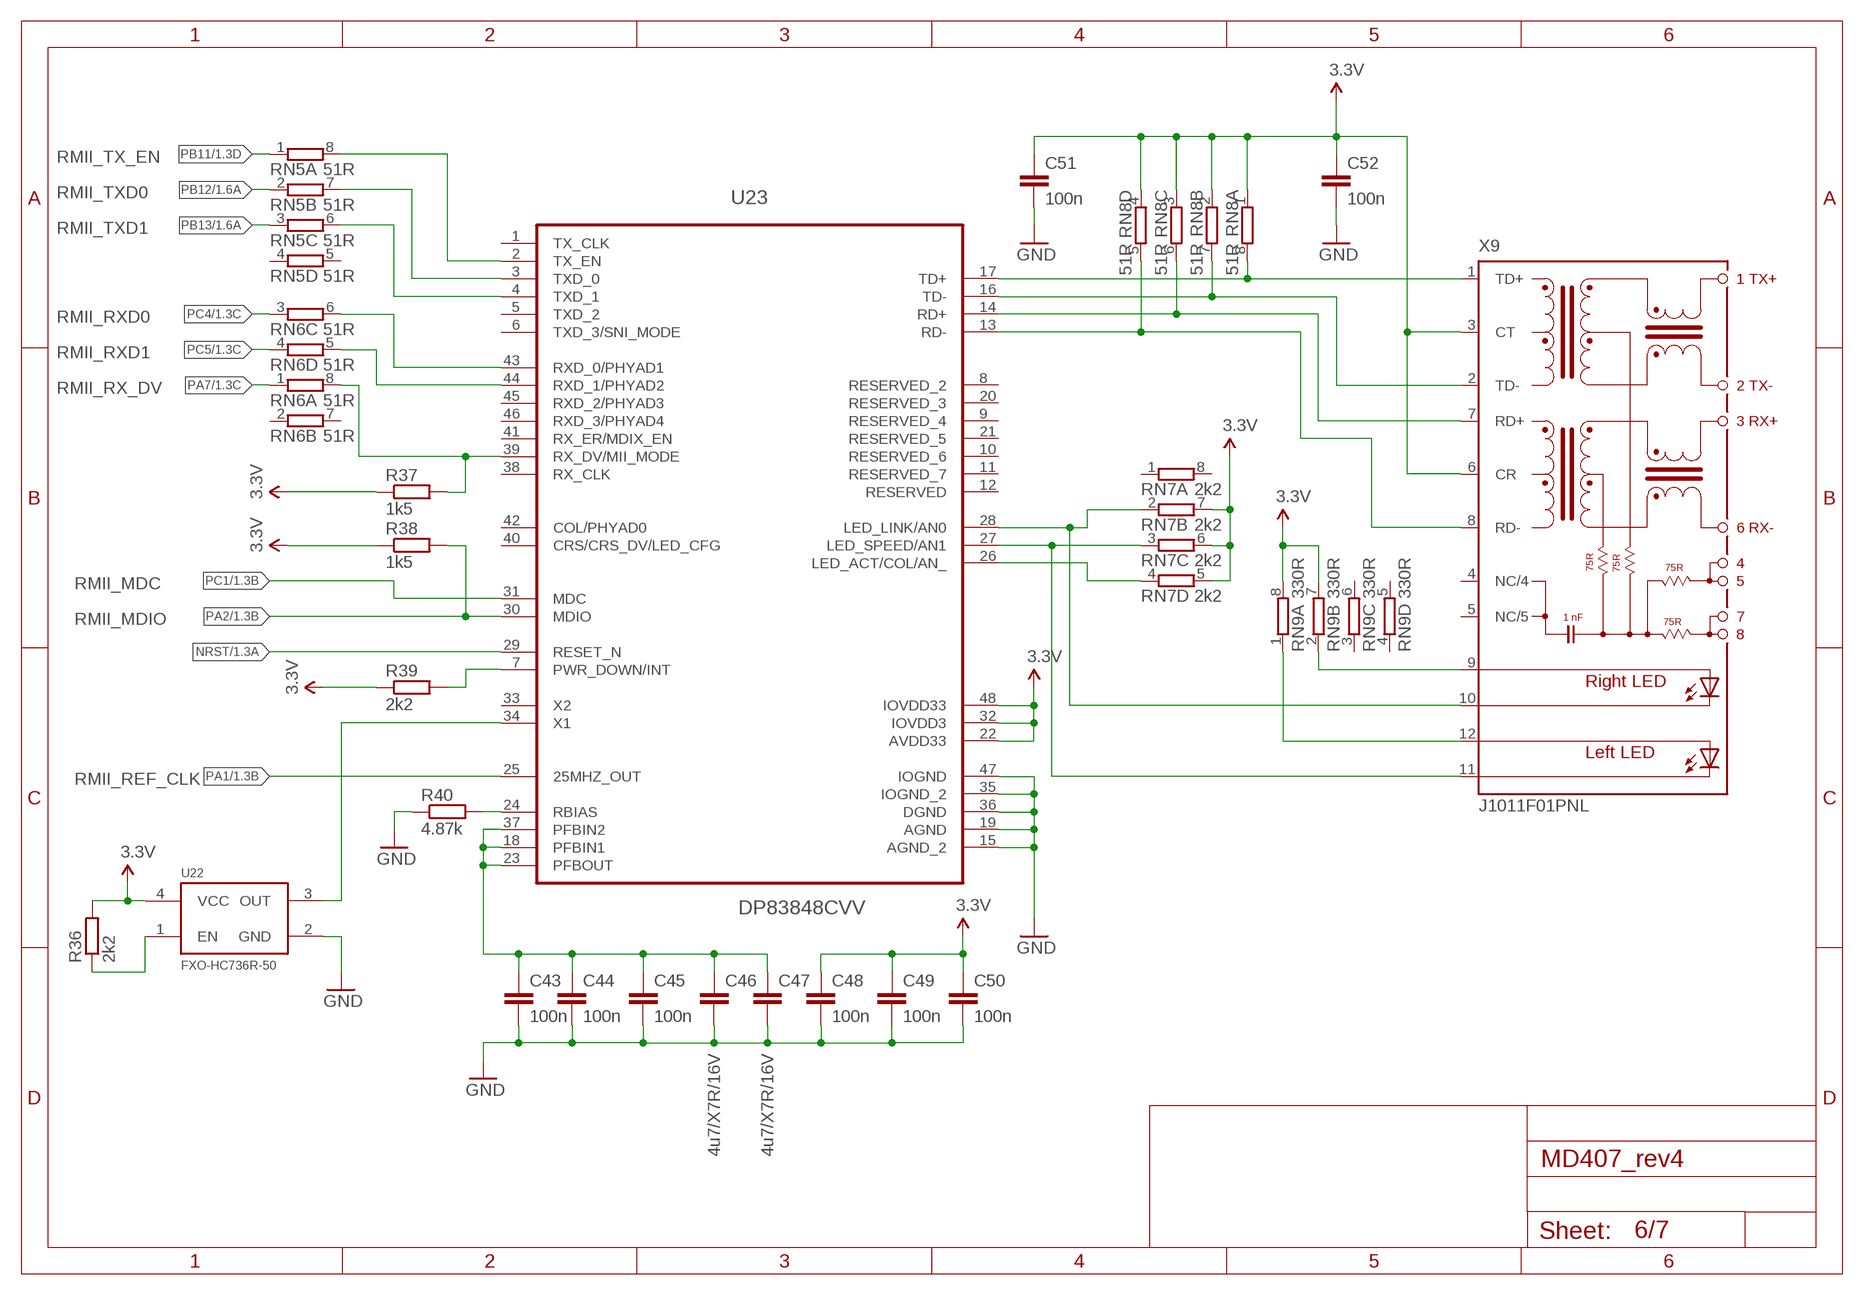
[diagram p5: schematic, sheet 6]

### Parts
C43  100n  C-EUC0603  [C0603]
C44  100n  C-EUC0603  [C0603]
C45  100n  C-EUC0603  [C0603]
C46  4u7/X7R/16V  C-EUC0805  [C0805]
C47  4u7/X7R/16V  C-EUC0805  [C0805]
C48  100n  C-EUC0603  [C0603]
C49  100n  C-EUC0603  [C0603]
C50  100n  C-EUC0603  [C0603]
C51  100n  C-EUC0603  [C0603]
C52  100n  C-EUC0603  [C0603]
R36  2k2  R-EU_R0603  [R0603]
R37  1k5  R-EU_R0603  [R0603]
R38  1k5  R-EU_R0603  [R0603]
R39  2k2  R-EU_R0603  [R0603]
R40  4.87k  R-EU_R0603  [R0603]
RN5  51R  4R-NCAY16  [CAY16]
RN6  51R  4R-NCAY16  [CAY16]
RN7  2k2  4R-NCAY16  [CAY16]
RN8  51R  4R-NCAY16  [CAY16]
RN9  330R  4R-NCAY16  [CAY16]
U22  FXO-HC736R-50  [CRYSTAL-SMD-7.5X5.2-6PIN]
U23  DP83848CVV  [QFP50P900X900X160-48N]
X9  J1011F01PNL  [J1]

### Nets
3.3V: C48.1 C49.1 C50.1 C51.1 C52.1 R36.2 R37.1 R38.1 R39.1 RN7.5 RN7.6 RN7.7 RN8.1 RN8.2 RN8.3 RN8.4 RN9.7 RN9.8 U22.4(VCC) U23.22(AVDD33) U23.32(IOVDD3) U23.48(IOVDD33) X9.3(CT) X9.6(CR) ; also sheet 1,2,3,4,5,7
GND: C43.2 C44.2 C45.2 C46.2 C47.2 C48.2 C49.2 C50.2 C51.2 C52.2 R40.1 U22.2(GND) U23.15(AGND_2) U23.19(AGND) U23.35(IOGND_2) U23.36(DGND) U23.47(IOGND) ; also sheet 1,2,3,4,5,7
N$12: R40.2 U23.24(RBIAS)
N$14: C43.1 C44.1 C45.1 C46.1 C47.1 U23.18(PFBIN1) U23.23(PFBOUT) U23.37(PFBIN2)
N$32: RN6.6 U23.43(RXD_0/PHYAD1)
N$33: RN5.8 U23.2(TX_EN)
N$37: RN6.5 U23.44(RXD_1/PHYAD2)
N$39: R37.2 RN6.8 U23.39(RX_DV/MII_MODE)
N$50: RN9.2 X9.9(A-R)
N$51: RN5.7 U23.3(TXD_0)
N$52: RN5.6 U23.4(TXD_1)
N$53: RN8.8 U23.17(TD+) X9.1(TD+)
N$54: RN8.7 U23.16(TD-) X9.2(TD-)
N$55: R39.2 U23.7(PWR_DOWN/INT)
N$57: RN7.2 U23.28(LED_LINK/AN0) X9.10(C-R)
N$58: RN7.3 U23.27(LED_SPEED/AN1) X9.11(C-L)
N$59: RN7.4 U23.26(LED_ACT/COL/AN_)
N$60: RN9.1 X9.12(AL)
N$79: RN8.6 U23.14(RD+) X9.7(RD+)
N$80: RN8.5 U23.13(RD-) X9.8(RD-)
N$82: U22.3(OUT) U23.34(X1)
N$83: R36.1 U22.1(EN)
NRST: U23.29(RESET_N) ; also sheet 1,2
PA1: U23.25(25MHZ_OUT) ; also sheet 1,2
PA2: R38.2 U23.30(MDIO) ; also sheet 1,2
PA7: RN6.1 ; also sheet 1,2
PB11: RN5.1 ; also sheet 1,2
PB12: RN5.2 ; also sheet 1,2
PB13: RN5.3 ; also sheet 1,2
PC1: U23.31(MDC) ; also sheet 1,2
PC4: RN6.3 ; also sheet 1,2
PC5: RN6.4 ; also sheet 1,2
Unconnected: RN5.4 RN5.5 RN6.2 RN6.7 RN7.1 RN7.8 RN9.3 RN9.4 RN9.5 RN9.6 U23.1(TX_CLK) U23.5(TXD_2) U23.6(TXD_3/SNI_MODE) U23.8(RESERVED_2) U23.9(RESERVED_4) U23.10(RESERVED_6) U23.11(RESERVED_7) U23.12(RESERVED) U23.20(RESERVED_3) U23.21(RESERVED_5) U23.33(X2) U23.38(RX_CLK) U23.40(CRS/CRS_DV/LED_CFG) U23.41(RX_ER/MDIX_EN) U23.42(COL/PHYAD0) U23.45(RXD_2/PHYAD3) U23.46(RXD_3/PHYAD4) X9.4(NC/4) X9.5(NC/5)

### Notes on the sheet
- RMII_TX_EN
- RMII_TXD0
- RMII_TXD1
- RMII_RXD0
- RMII_RXD1
- RMII_RX_DV
- RMII_MDC
- RMII_MDIO
- RMII_REF_CLK

## Sheet 7 of 7: CAN
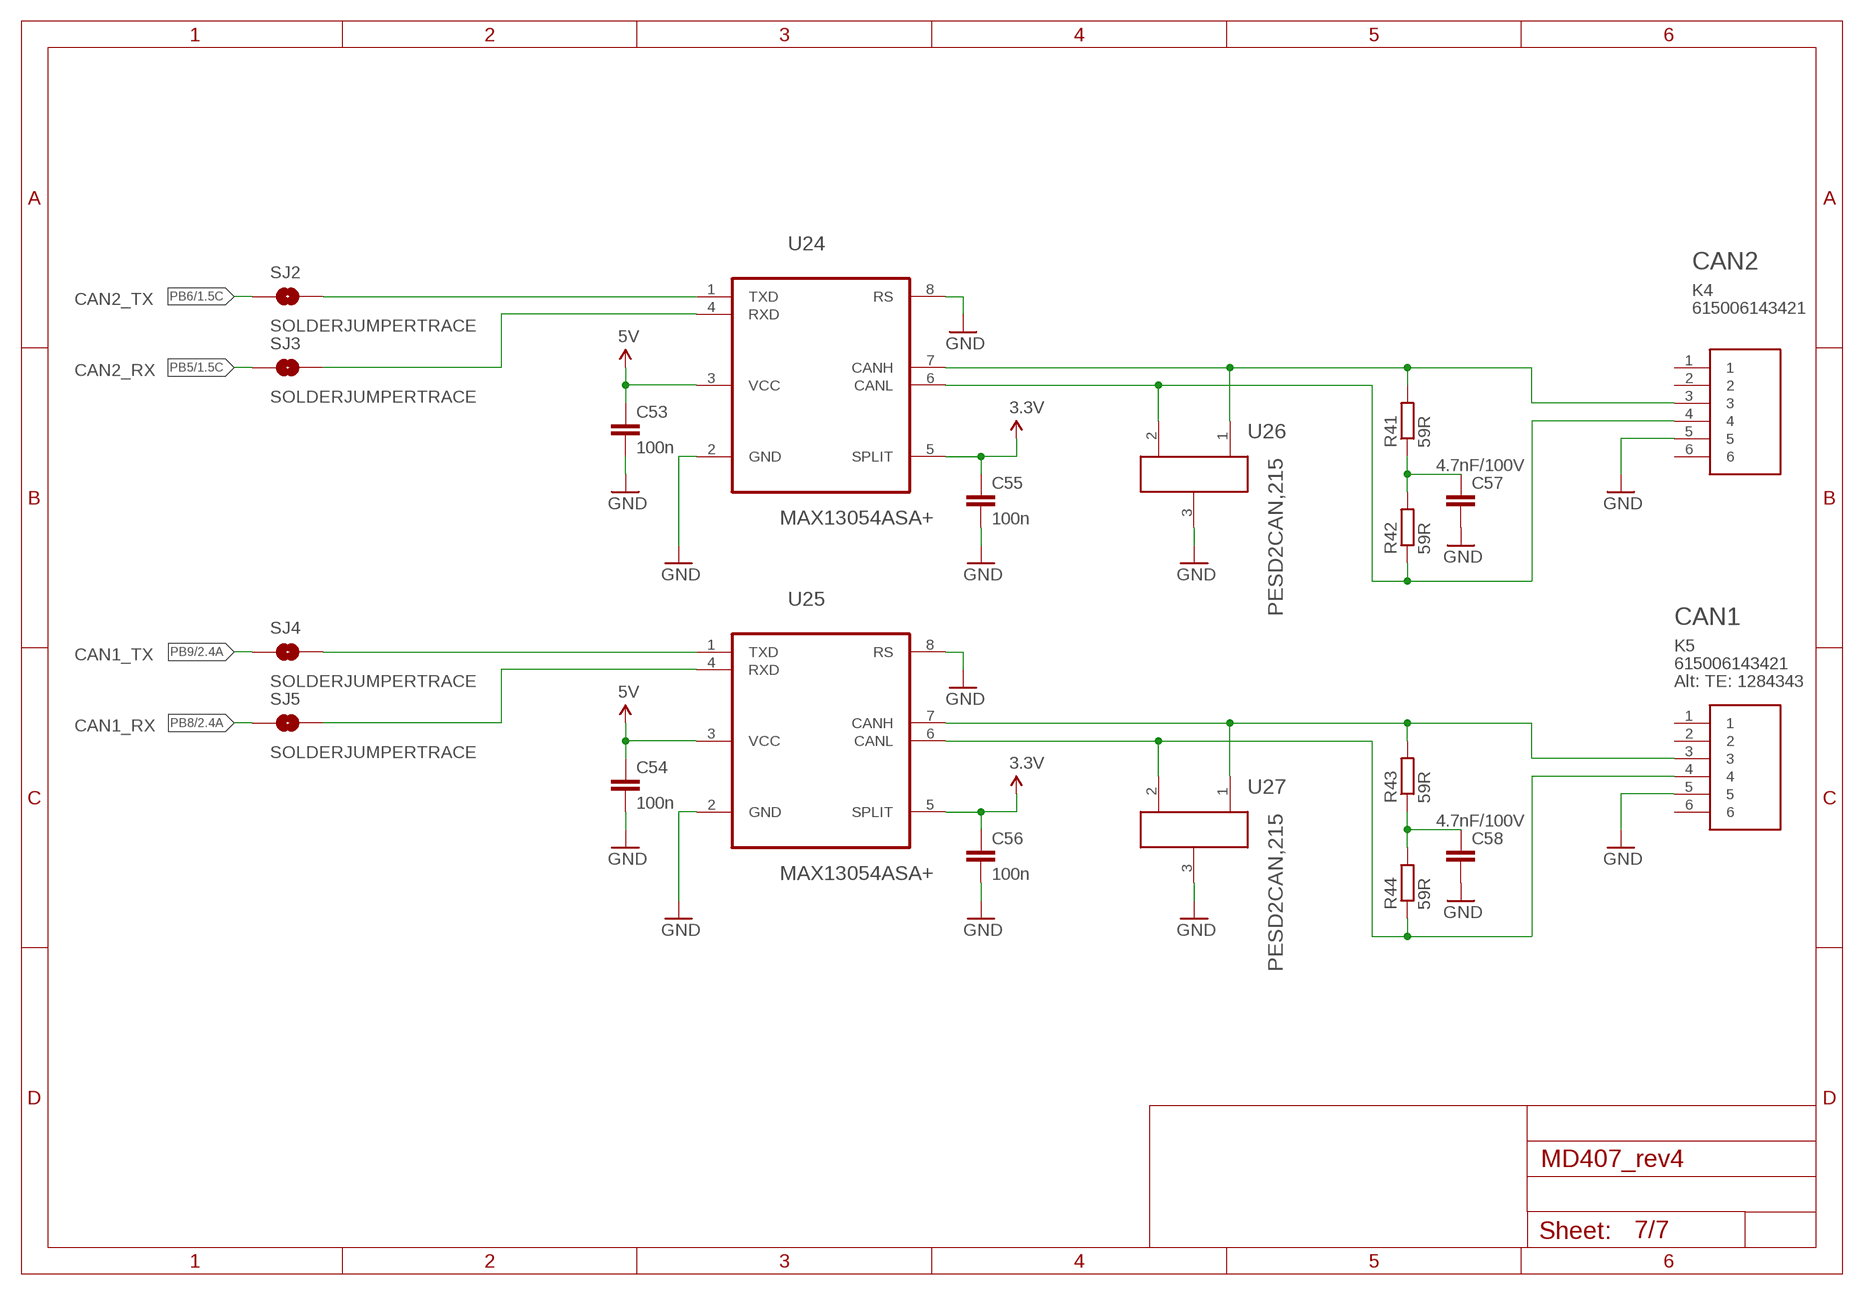
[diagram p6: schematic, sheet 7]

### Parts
C53  100n  C-EUC0603  [C0603]
C54  100n  C-EUC0603  [C0603]
C55  100n  C-EUC0603  [C0603]
C56  100n  C-EUC0603  [C0603]
C57  4.7nF/100V  C-EUC0805  [C0805]
C58  4.7nF/100V  C-EUC0805  [C0805]
K4  615006143421  [615006143421]
K5  615006143421  [615006143421]
R41  59R  R-EU_R0603  [R0603]
R42  59R  R-EU_R0603  [R0603]
R43  59R  R-EU_R0603  [R0603]
R44  59R  R-EU_R0603  [R0603]
SJ2  SOLDERJUMPERTRACE  [SJ_2S-TRACE]
SJ3  SOLDERJUMPERTRACE  [SJ_2S-TRACE]
SJ4  SOLDERJUMPERTRACE  [SJ_2S-TRACE]
SJ5  SOLDERJUMPERTRACE  [SJ_2S-TRACE]
U24  MAX13054ASA+  [SOIC127P600X175-8N]
U25  MAX13054ASA+  [SOIC127P600X175-8N]
U26  PESD2CAN,215  [SOT23]
U27  PESD2CAN,215  [SOT23]

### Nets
3.3V: C55.1 C56.1 U24.5(SPLIT) U25.5(SPLIT) ; also sheet 1,2,3,4,5,6
5V: C53.1 C54.1 U24.3(VCC) U25.3(VCC) ; also sheet 2,3,4,5
GND: C53.2 C54.2 C55.2 C56.2 C57.2 C58.2 K4.5 K5.5 U24.2(GND) U24.8(RS) U25.2(GND) U25.8(RS) U26.3 U27.3 ; also sheet 1,2,3,4,5,6
N$26: K4.4 R42.1 U24.6(CANL) U26.2
N$29: K4.3 R41.2 U24.7(CANH) U26.1
N$64: K5.4 R44.1 U25.6(CANL) U27.2
N$65: C58.1 R43.1 R44.2
N$66: C57.1 R41.1 R42.2
N$67: SJ2.2 U24.1(TXD)
N$68: SJ3.2 U24.4(RXD)
N$88: K5.3 R43.2 U25.7(CANH) U27.1
N$93: SJ4.2 U25.1(TXD)
N$94: SJ5.2 U25.4(RXD)
PB5: SJ3.1 ; also sheet 1,2
PB6: SJ2.1 ; also sheet 1,2
PB8: SJ5.1 ; also sheet 1,2
PB9: SJ4.1 ; also sheet 1,2
Unconnected: K4.1 K4.2 K4.6 K5.1 K5.2 K5.6

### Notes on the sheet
- CAN2
- CAN2_TX
- CAN2_RX
- CAN1
- CAN1_TX
- Alt: TE: 1284343
- CAN1_RX

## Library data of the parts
C1-C8 C10-C28 C30 C31 C33-C42 = rcl:C-EU: CAPACITOR, European symbol
C9 C29 C32 C43-C58 = resistor:C-EU: CAPACITOR, European symbol
D1 = diode:SMF5.0AT1: 200 W Transient Voltage Suppressor
D2 = diode:DIODE-: DIODE
F1 = MD407:1812L050PR: Resettable PTC
F2 = MD407:1812L020PR: Resettable PTC
H1-H6 = holes:MOUNT-HOLE: MOUNTING HOLE with drill center marker
JP1 = pinhead:PINHD-2X3: PIN HEADER
K1 = USBSteckverbinderWR-COM:61400416121: WR-COM Horizontal USB Type B
K2 = USBSteckverbinderWR-COM:61400416021: WR-COM Horizontal USB Type A
K3 = MD407:FC681465P
K4 K5 = ModularJackliegendhalb-geschirmtWR-MJ:615006143421: WR-MJ Horizontal 6P6C Half Shielded Modular Jack Tab Down, 6 Pins
L1 = WE-PD:WE-PD: SMD-Shielded Power Inductors WE-PD; MPN: 7447789118; OC_FARNELL: 2082719; OC_NEWARK: 88T7170; PACKAGE: 7332; SUPPLIER: Wuerth Elektronik
LED1 LED2 = MD407:LED: LEDs
LED3-LED7 = SparkFun-LED:LED: LEDs
R1-R4 R6 R7 R9 R11 R17-R40 = rcl:R-EU_: RESISTOR, European symbol
R5 R8 R10 R12-R16 R41-R44 = resistor:R-EU_: RESISTOR, European symbol
RN1-RN9 = resistor-dil:4R-N: Array Chip Resistor Source: RS Component / Phycomp; OC_FARNELL: unknown; OC_NEWARK: unknown
S1 S2 = STM32_devboard:SKQBARA010
SJ1-SJ5 = SparkFun-Passives:SOLDERJUMPER: Solder Jumper
SW1 = MD407:25436NAH: SWITCH, SPDT, 1A, 30VDC, THT; MPN: 25436NAH; OC_FARNELL: 1607954
U1 = STM32_devboard:STM32F407VGT7: STmicroelectronics Cortex M4 Series Typ: STM32F407Vx LQFP100 Copyright 2012 by Ersan Günes, Quantitec, info@quantitec.de
U2-U12 = STM32_devboard:TPD8F003
U13 = MD407:500901-0801: Memory Card Connectors RIGHT ANGLE; SUPPLIER: Molex
U14 = STM32_devboard:TPA6111A2D: AUDIO POWER AMPLIFIER; MPN: TPA6111A2D; OC_FARNELL: 8456593; OC_NEWARK: 38K8607; PACKAGE: SOIC-8; SUPPLIER: TI
U15 U16 = STM32_devboard:SP3003-02JTG: 0.65pF Rail Clamp Array; MPN: SP3003-02JTG; OC_FARNELL: 1827640; OC_NEWARK: 31T1604; PACKAGE: SC70-5; SUPPLIER: LITTELFUSE
U17 = STM32_devboard:STMPS2141STR
U18 = STM32_devboard:FT230XS: I/F, USB2.0 FS TO BASIC UART; MPN: FT230XS; OC_FARNELL: 2081321; OC_NEWARK: 83T7087; PACKAGE: SSOP-16; SUPPLIER: FTDI
U19 = STM32_devboard:DF01S: Bridge Rectifiers; MPN: DF01S; OC_FARNELL: 1470959; OC_NEWARK: 84K0208; PACKAGE: SDIP-4; SUPPLIER: Fairchild
U20 = STM32_devboard:LP3875EMP-3.3: Linear Regulator; MPN: LP3875EMP-3.3; OC_FARNELL: 1685728; OC_NEWARK: 41K7593; PACKAGE: SOT223-5; SUPPLIER: NationalSemiconductor; VALUE: >VALUE
U21 = STM32_devboard:TPS54160ADGQ: 1.5-A, 60-V, Step-Down SWIFT DC/DC Converter with Eco-mode,MSOP-10; MPN: TPS54160ADGQ; OC_FARNELL: 2144283; OC_NEWARK: 27W5388; PACKAGE: MSOP-10; SUPPLIER: TEXAS INSTRUMENTS
U22 = MD407:FXO-HC736R-50: Generic 5x3 and 7x5 oscillators
U23 = STM32_devboard:DP83848CVV: Single Port 10/100 Mb/s Ethernet Physical Layer Transceiver; MPN: DP83848CVVX; OC_FARNELL: 1685784; PACKAGE: QFP-48; SUPPLIER: National Semiconductors
U24 U25 = STM32_devboard:MAX13054ASA+: Industry-Standard High-Speed CAN Transceivers with ±80V Fault Protection; MPN: MAX13054ASA+; OC_FARNELL: 1600117; OC_NEWARK: 99K2881; PACKAGE: SOIC-8; SUPPLIER: Maxim
U26 U27 = STM32_devboard:PESD2CAN,215
U$1-U$3 = STM32_devboard:FIDUCIAL: For use by pick and place machines to calibrate the vision/machine, 1mm
X1 X6 = STM32_devboard:61205021621
X2 = STM32_devboard:61202021621: CONNECTOR 20-pin series 057 contact pc board low profile headers
X3-X5 X7 = STM32_devboard:61201021621
X8 = con-lumberg_temp2:KLBR4: Jack connectors according to JISC 6560, 3.5 mm Klinkeneinbaukupplung nach JISC 6560, 3,5 mm, 3-polig/ stereo, abgewinkelte Ausführung, mit Öffner, für Leiterplatten Source: Data sheet; MPN: KLBR 4; OC_FARNELL: 1217016; OC_NEWARK: 97K2709
X9 = STM32_devboard:J1011F: PULSEJACK (TM) 1x1 Tab-UP RJ45 10/100 Base-TX RJ45 1x1 Tab-UP with LEDs 8-pin (J1 series) and 6-pin (JP series) integrated magnetics connector, designed to support applications, such as ADSL modems, LAN-on-Motherboard, and Hub and Switches. Source: www.pulseeng.com .. PulseJack-J402.pdf
Y1 = STM32_devboard:7B-8.000MAAJ-T

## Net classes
1 HP: width 0.762 mm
